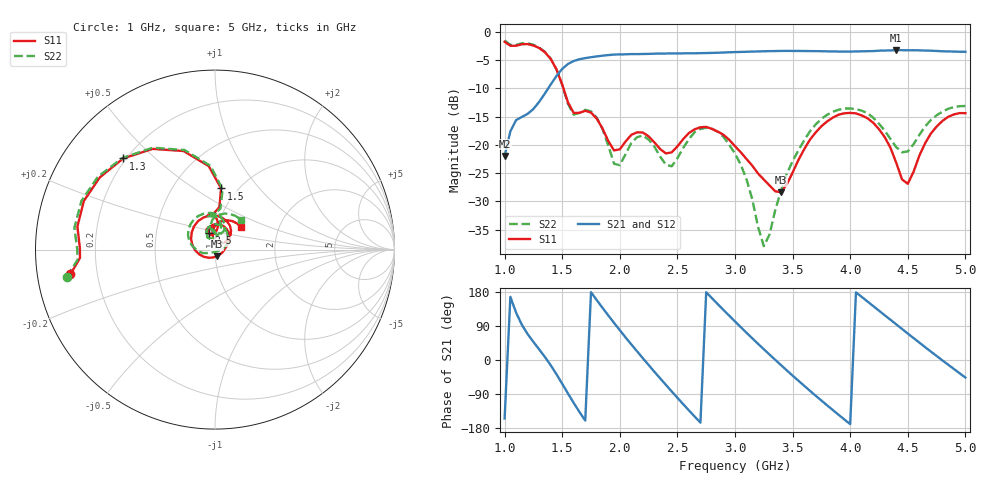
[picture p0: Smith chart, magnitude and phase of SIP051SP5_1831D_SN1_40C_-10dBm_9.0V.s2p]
# GHz  S  dB  R  50
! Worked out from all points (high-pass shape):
!   81 points, 1 GHz to 5 GHz, reference 50 ohm
!   highest |S21| = -3.23 dB at 4.4 GHz (marker M1); lowest = -22.0 dB at 1 GHz (marker M2)
!   |S21| within 3 dB of the highest: 1.519 GHz to end of sweep
!   lowest |S11| = -28.4 dB at 3.4 GHz (marker M3), VSWR 1.08, Z = 50.9 - j3.74 ohm
!   |S11| at or under -10 dB: 1.511 GHz to end of sweep
!   |S22| runs from -37.9 to -1.5 dB; largest |S21 - S12| = 0.0027
!   S11 on the Smith chart (normalised r, x): 1 GHz: 0.10, -0.08; 1.3 GHz: 0.19, +0.40; 1.5 GHz: 0.84, +0.65; 2.5 GHz: 0.92, +0.17; 5 GHz: 1.29, +0.33
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1  -1.75 -170.3  -21.99 -154.4  -21.98 -154.2  -1.52 -169.7
1.1  -2.46 179.2  -15.61 124.8  -15.64 124.7  -2.30 180.0
1.3  -2.85 135.2  -12.39 28.1  -12.40 28.1  -2.79 135.3
1.5  -9.31 84.3  -6.56 -62.7  -6.56 -62.6  -9.41 82.8
1.6  -14.37 95.0  -5.16 -113.4  -5.14 -113.4  -14.66 94.4
1.7  -13.97 100.1  -4.64 -159.7  -4.65 -159.8  -13.79 100.2
1.85  -17.11 82.4  -4.22 137.7  -4.21 137.6  -17.21 75.0
2  -20.80 110.4  -3.99 78.6  -3.98 78.7  -23.61 112.0
2.2  -17.82 99.6  -3.91 4.6  -3.91 4.6  -18.35 102.9
2.35  -20.74 91.7  -3.85 -48.3  -3.85 -48.3  -22.07 89.0
2.5  -20.28 110.2  -3.82 -99.7  -3.81 -99.8  -22.37 121.6
2.75  -16.82 77.8  -3.75 178.8  -3.75 178.8  -16.99 87.7
3  -20.24 35.3  -3.58 101.7  -3.58 101.8  -21.54 32.6
3.25  -26.14 -5.8  -3.44 28.4  -3.43 28.4  -37.94 -70.9
3.4  -28.37 -73.9  -3.38 -13.7  -3.38 -13.7  -28.08 -152.9
3.7  -17.82 168.5  -3.41 -94.2  -3.41 -94.1  -16.40 161.2
4.05  -14.43 87.9  -3.46 178.6  -3.47 178.6  -13.68 97.9
4.35  -20.53 36.9  -3.28 106.1  -3.29 106.0  -18.97 65.0
4.4  -23.21 36.7  -3.23 94.0  -3.24 94.0  -20.42 69.3
4.5  -26.90 74.9  -3.26 69.8  -3.24 69.8  -21.17 88.9
4.7  -18.01 92.0  -3.34 22.3  -3.34 22.4  -15.61 95.3
5  -14.40 40.3  -3.53 -46.3  -3.52 -46.3  -13.12 49.3
